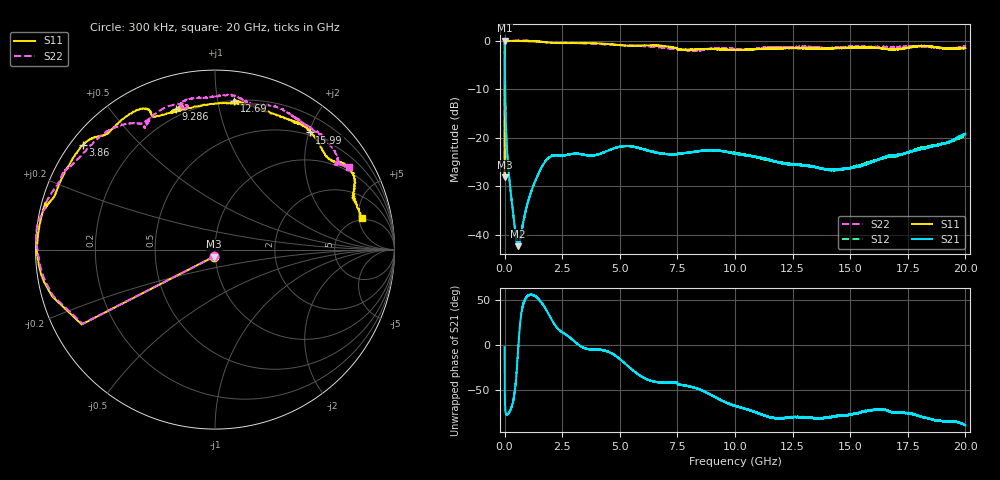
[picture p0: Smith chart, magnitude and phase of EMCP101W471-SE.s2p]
!EMCP101W471
!Johanson Technology Inc.
!www.johansontechnology.com
!Test Board Conditions:
!Substrate Type  RO4350B
!Substrate Thickness  10 mil
!Substrate Dk  3.66
!TL Type: GCPW
!TL Trace Width  20 mil
!TL Gap  10 mil
!PART MODE SINGLE ENDED (AKA BYPASS)
!DUT TOPOLOGY	SERIES-SHUNT
# MHz S  dB  R 50
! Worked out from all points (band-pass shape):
!   20001 points, 300 kHz to 20 GHz, reference 50 ohm
!   highest |S21| = -0.01 dB at 300 kHz (marker M1); lowest = -42.3 dB at 580.3 MHz (marker M2)
!   |S21| within 3 dB of the highest: start of sweep to 7.352 MHz
!   lowest |S11| = -28.2 dB at 300 kHz (marker M3), VSWR 1.08, Z = 49.4 - j3.82 ohm
!   |S11| at or under -10 dB: start of sweep to 2.558 MHz
!   |S22| runs from -28.4 to 0.0 dB; largest |S21 - S12| = 0.0058
!   S11 on the Smith chart (normalised r, x): 300 kHz: 0.99, -0.08; 3.86 GHz: 0.04, +0.35; 9.286 GHz: 0.16, +0.75; 12.69 GHz: 0.20, +1.12; 15.99 GHz: 0.45, +2.01; 20 GHz: 4.63, +5.50
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0.3  -28.20 -96.9  -0.01 -2.3  -0.01 -2.5  -28.39 -95.1
105.298  -0.10 -176.8  -22.43 -77.4  -22.41 -77.5  -0.17 -176.3
166.298  -0.04 -179.0  -26.52 -76.2  -26.45 -76.3  -0.14 -178.6
274.296  -0.06 178.9  -31.68 -71.0  -31.65 -71.0  -0.08 179.6
580.291  -0.09 174.5  -42.34 -6.8  -42.34 -7.4  -0.01 176.2
1137.283  -0.14 168.1  -31.33 56.1  -31.35 56.2  -0.05 170.1
1754.274  -0.33 164.6  -25.02 41.7  -24.94 41.7  -0.34 160.4
3334.25  -0.54 147.7  -23.42 -1.9  -23.41 -1.8  -0.54 151.4
3860.242  -0.55 141.6  -23.66 -5.0  -23.64 -4.8  -0.67 149.3
5229.222  -1.06 133.8  -21.71 -20.5  -21.76 -20.2  -0.95 134.8
6667.2  -1.03 118.2  -23.17 -41.4  -23.13 -41.8  -1.38 124.7
7600.186  -1.83 113.2  -23.28 -44.0  -23.28 -43.9  -1.81 116.6
8379.174  -1.79 103.8  -22.84 -48.6  -22.79 -48.9  -2.07 119.8
9286.161  -1.79 105.6  -22.65 -60.1  -22.72 -59.4  -1.52 108.8
10000.15  -1.97 106.0  -23.28 -67.6  -23.12 -67.2  -1.75 101.2
11342.13  -1.69 81.4  -24.36 -79.0  -24.47 -79.0  -1.46 101.6
12692.11  -1.56 82.6  -25.59 -80.0  -25.51 -80.2  -1.33 88.3
13334.1  -1.68 76.3  -25.89 -81.1  -25.88 -81.2  -1.36 81.0
14406.08  -1.59 59.6  -26.59 -79.2  -26.66 -79.1  -1.50 72.9
15992.06  -1.52 51.0  -24.96 -72.2  -24.80 -73.7  -1.33 58.7
16667.05  -1.80 42.2  -23.70 -73.6  -23.98 -74.0  -1.32 56.4
20000  -1.54 12.2  -19.19 -89.4  -19.51 -87.7  -1.11 31.5
